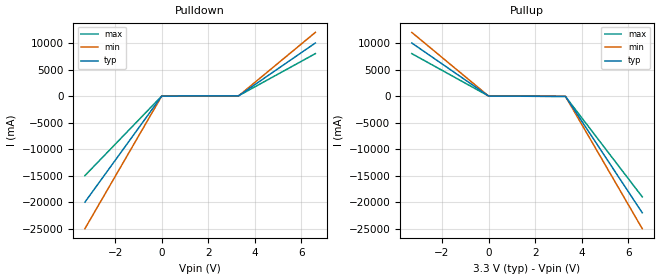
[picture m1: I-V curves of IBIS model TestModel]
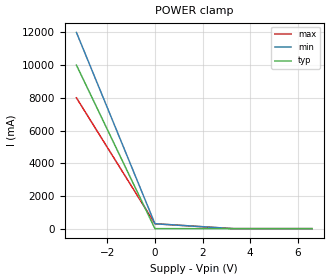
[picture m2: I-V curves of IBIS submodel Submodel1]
|DESCRIPTION OF BUG:
|"Dangling" models, present but not referenced or used in the file, are not
|flagged to the user.  These include [Model]s which are not described in
|[Pin], [Model Selector] or [Driver Schedule] sections and also [Submodel]s
|which are not referenced by any [Add Submodel] declaration.
|Some indication -- most appropriately, a warning -- should be made of the
|lack of reference for these models and model fragments.
|An example:
|  WARNING (line  xxx) - Model xxx not referenced in [Pin], [Model Selector]
|  or [Driver Schedule] sections.
|For Submodels:
|  WARNING (line  xxx) - Submodel xxx not referenced by [Add Submodel]
|  keyword.
|This bug also applies to DOS32 IBISCHK3 v3.2.5.
|ADDITIONAL NOTES:
|As pointed out by Mike LaBonte of Cadence, this BUG should also apply to
|[Model]s which are not referenced in a [Series Pin Mapping] section.
|Therefore, a "dangling" [Model] is one which, while syntactically correct,
|is not referenced in [Pin], [Model Selector], [Driver Schedule] or [Series
|Pin Mapping] sections.
|Ian Dodd of Cadence raised the point that, for devices such as an FPGA, an
|unreferenced [Model] may be desirable in a user-ready model (such a [Model]
|might represent a available programming option which may or may not be
|implemented after the user configures the device).  In addition, generating
|a message for every instance of an unreferenced [Model] may be unnecessarily
|confusing to the user.
|To address the above, the following changed messages are proposed:
|For one or more instances of an unreferenced [Model]:
|  WARNING (line  xxx) - [Model] zzz not referenced in [Pin],
|  [Model Selector], [Driver Schedule] or [Series Pin Mapping] sections.
|Only one instance of the above warning message should be generated, for
|the first unreferenced [Model] in the file.  Multiple unreferenced [Model]s
|in an IBIS file should NOT generate multiple warning messages.
|For Submodels:
|  WARNING (line  xxx) - [Submodel] zzz not referenced by [Add Submodel]
|  keyword.
|As [Submodel]s should not exist independently of a referencing [Add
|Submodel]
|keyword, the above message should be generated for EVERY instance of
|an unreferenced [Submodel].
[IBIS Ver]   3.2
[File Name]   bug49.ibs
[File Rev]   0.0
[Date]   02-November-2000
[Source]   File created from specification
[Disclaimer]
   (C) Copyright 2000 Intel Corp.
   All rights reserved
   This model is for demonstration purposes only.
[Component]   GENERIC_IBIS
[Manufacturer]   Intel Corp.
[Package]
|   typ   min   max
R_pkg   6.0mO   5.0mO   7.0mO
L_pkg   5.0nH   2.0nH   8.0nH
C_pkg   1.0pF   0.5pF   1.5pF
[Pin]   signal_name   model_name   R_pin   L_pin   C_pin
   A1   TestSignal1   TestModel
   A2   TestSignal2   TestModel
| Models and submodels in the file (5): TestModel (Output), TestModel2 (Output), TestModel3 (Output), Submodel1 (Dynamic_clamp), Submodel2 (Dynamic_clamp)
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[Model]   TestModel
Model_type   Output
Polarity   Non-Inverting
Cref = 10.0pF
C_comp   5.00pF   4.00pF   6.00pF
[Temperature Range]   27.00   100.00   0.00
[Voltage Range]   3.30V   3.00V   3.60V
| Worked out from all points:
|   slope of the pulldown table from 0 to 0.495 V, typ, clamps not added: 82.5 ohm
|   slope of the pullup table from 0 to 0.495 V, typ, clamps not added: 50.8 ohm
[Pulldown]
| voltage   I(typ)   I(min)   I(max)
-3.3V     -20A       -25A       -15A
0V        0A         -5nA       5nA
3.3V      40mA       32mA       48mA
6.6V      10A        12A        8A
[Pullup]
| voltage   I(typ)   I(min)   I(max)
-3.3V     10A        12A        8A
0V        0A         -300nA     300nA
3.3V      -65mA      -40mA      -80mA
6.6V      -22A       -25A       -19A
[Ramp]
| variable   typ   min   max
dV/dt_r   0.35/1.6n   0.25/1.8n   0.45/1.5n
dV/dt_f   0.35/1.6n   0.25/1.8n   0.45/1.5n
R_load = 50.000
[Submodel] Submodel1
Submodel_type  Dynamic_clamp
[Power Clamp]
| voltage   I(typ)   I(min)   I(max)
-3.3V     10A        12A        8A
0V        0A         300mA      300mA
3.3V      0A         0A         0A
6.6V      0A         0A         0A
